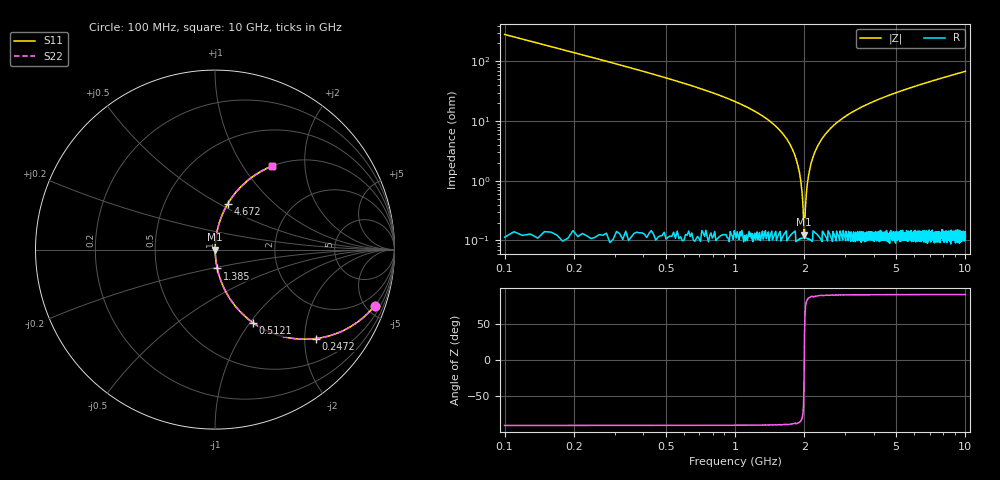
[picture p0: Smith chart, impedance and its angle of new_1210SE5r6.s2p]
!	AVX	Thin	Film	Operation	Date:	April 2007
!	Description:	Accu-P®	"Series,"	Thin	"Film,"	"SMD,"	RF	Capacitor
!	Part	Number:	1210J5R6ABT
!	100	MHz	-	5.05	GHz
!	Serial	Measurements
#	MHZ	S	MA	R	50
!	S11	S21	S12	S22
!	dB	Phase	dB	Phase	dB	Phase	dB	Phase
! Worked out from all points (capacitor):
!   1010 points, 100 MHz to 10 GHz, reference 50 ohm
!   read as one part in series: C = 5.6 pF near 149.1 MHz
!   lowest |Z| = 126 mohm at 1.994 GHz (marker M1)
!   series resonance near 1.998 GHz, so ESL is about 1.1 nH
!   S11 on the Smith chart (normalised r, x): 100 MHz: 1.00, -5.67; 247.2 MHz: 1.00, -2.26; 512.1 MHz: 1.00, -1.04; 1.385 GHz: 1.00, -0.21; 4.672 GHz: 1.00, +0.54; 10 GHz: 1.00, +1.37
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100  0.943 -19.4  0.333 70.5  0.333 70.5  0.943 -19.4
247.175  0.749 -41.4  0.662 48.5  0.662 48.5  0.749 -41.4
512.091  0.46 -62.5  0.887 27.4  0.887 27.4  0.46 -62.5
835.877  0.27 -74.1  0.962 15.7  0.962 15.7  0.27 -74.1
1385.332  0.106 -83.3  0.993 6.1  0.993 6.1  0.106 -83.3
1758.176  0.036 -86.0  0.998 2.1  0.998 2.1  0.036 -86.0
1885.728  0.016 -84.9  0.999 0.9  0.999 0.9  0.016 -84.9
1924.975  0.011 -82.9  0.999 0.6  0.999 0.6  0.011 -82.9
1964.222  0.00498 -75.8  0.999 0.3  0.999 0.3  0.00498 -75.8
1993.657  0.00134 -26.7  0.999 0.0  0.999 0.0  0.00134 -26.7
2032.904  0.00508 76.1  0.999 -0.3  0.999 -0.3  0.00508 76.1
2081.962  0.012 83.5  0.999 -0.7  0.999 -0.7  0.012 83.5
2131.021  0.018 85.2  0.999 -1.1  0.999 -1.1  0.018 85.2
2219.326  0.03 86.0  0.998 -1.7  0.998 -1.7  0.03 86.0
2337.066  0.045 85.9  0.998 -2.6  0.998 -2.6  0.045 85.9
2749.158  0.092 84.0  0.995 -5.3  0.995 -5.3  0.092 84.0
3406.541  0.157 80.5  0.986 -9.0  0.986 -9.0  0.157 80.5
4672.25  0.262 74.6  0.964 -15.2  0.964 -15.2  0.262 74.6
5054.906  0.29 72.9  0.956 -16.9  0.956 -16.9  0.29 72.9
6703.271  0.398 66.4  0.916 -23.5  0.916 -23.5  0.398 66.4
8351.635  0.489 60.6  0.871 -29.2  0.871 -29.2  0.489 60.6
10000  0.564 55.6  0.825 -34.3  0.825 -34.3  0.564 55.6
